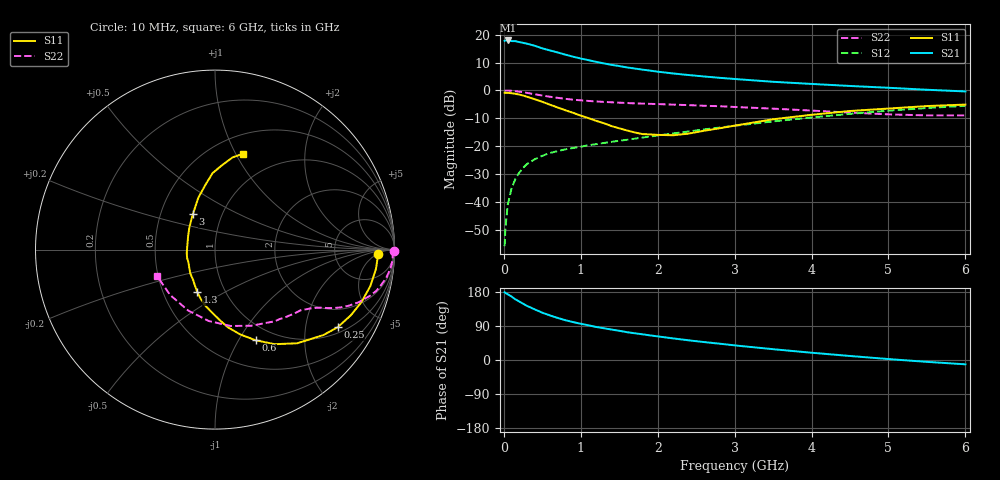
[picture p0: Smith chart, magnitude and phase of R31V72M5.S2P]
! SIEMENS Small Signal Semiconductors
! BFR181
! Si NPN RF Bipolar Junction Transistor in SOT23
! VCE = 1.75 V  IC = 2.5 mA
! Common Emitter S-Parameters:  May  1996
# GHz  S  MA  R  50
!  f  S11  S21  S12  S22
! GHz  MAG  ANG  MAG  ANG  MAG  ANG  MAG  ANG
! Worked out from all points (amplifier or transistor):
!   36 points, 10 MHz to 6 GHz, reference 50 ohm
!   highest |S21| = 17.9 dB at 50 MHz (marker M1)
!   |S21| within 3 dB of that: start of sweep to 521.7 MHz
!   unconditionally stable (mu >= 1): 1.43 GHz to 3.293 GHz
!   at 250 MHz: K = 0.27, MSG = 22.4 dB, |S12| = -27.8 dB
!   at 1.4 GHz: K = 0.99, MSG = 13.8 dB, |S12| = -18.5 dB
!   at 6 GHz: K = 0.86, MSG = 2.6 dB, |S12| = -5.5 dB
!   S11 on the Smith chart (normalised r, x): 10 MHz: 19, -5; 250 MHz: 1.21, -3.01; 600 MHz: 0.81, -1.18; 1.3 GHz: 0.74, -0.38; 3 GHz: 0.73, +0.30; 6 GHz: 0.69, +1.07
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0.01  0.9078 -1.4  7.751 178.9  0.0016 88.3  0.9963 -0.6
0.02  0.9076 -2.8  7.853 177.1  0.0033 90.9  0.9897 -1.2
0.05  0.9029 -6.9  7.869 173.6  0.0088 87.0  0.9921 -3.2
0.1  0.8891 -13.2  7.678 167.4  0.0174 82.1  0.9828 -6.2
0.15  0.8666 -19.8  7.638 160.0  0.0258 78.3  0.9675 -9.3
0.25  0.8089 -32.3  7.122 148.6  0.0408 71.5  0.927 -14.4
0.3  0.7687 -38.3  6.894 142.8  0.0475 69.5  0.9021 -16.5
0.4  0.6946 -48.7  6.33 133.7  0.0579 64.4  0.8529 -20.1
0.5  0.6236 -57.7  5.675 124.8  0.067 61.1  0.8075 -22.8
0.6  0.5533 -65.9  5.21 117.6  0.0752 58.7  0.7691 -24.8
0.7  0.4934 -73.4  4.792 111.0  0.0815 57.4  0.7344 -26.3
0.8  0.4396 -80.5  4.376 105.0  0.0874 56.2  0.7052 -27.5
0.9  0.3958 -85.9  4.022 100.0  0.0926 55.5  0.6803 -28.4
1.1  0.3183 -99.5  3.485 91.5  0.1035 55.1  0.6464 -30.2
1.3  0.2576 -112.3  3.047 83.8  0.1139 55.2  0.621 -31.9
1.6  0.1911 -136.2  2.584 73.4  0.1299 56.3  0.5932 -34.5
2.2  0.1565 169.4  2.012 57.0  0.1688 57.3  0.5549 -41.3
3  0.2327 122.0  1.601 38.6  0.2316 55.6  0.504 -53.6
3.5  0.3031 107.9  1.426 28.5  0.2772 52.7  0.4699 -64.6
4.5  0.4265 91.8  1.2 10.6  0.3792 43.6  0.3991 -95.1
5.5  0.5229 79.2  1.026 -4.9  0.4826 31.0  0.3557 -134.6
6  0.5565 73.7  0.957 -11.4  0.5286 23.7  0.3555 -155.8
